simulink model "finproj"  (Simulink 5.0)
settings: Solver=ode45  StartTime=0.0  StopTime=100.0  RelTol=1e-3
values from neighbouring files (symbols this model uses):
  denp = (abs(denp)>1e-8).*denp    [segway.m]
  nump = [nump 0]/numv(2)    [segway.m]

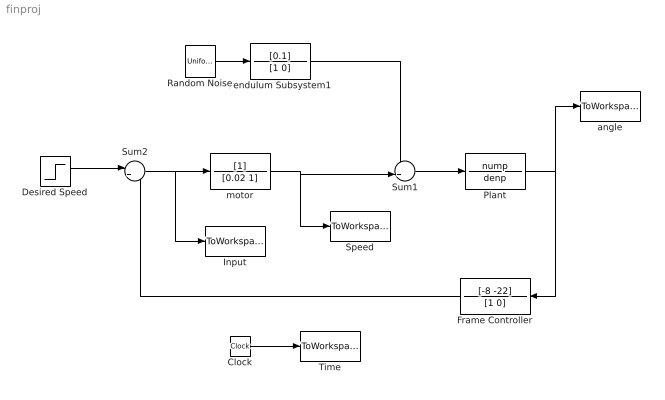
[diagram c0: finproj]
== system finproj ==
  Clock : Clock
  Desired Speed : Step  Time=0  After=0  SampleTime=0
  Frame Controller : TransferFcn  Orientation=left  Numerator=[-8 -22]  Denominator=[1 0]
  Input : ToWorkspace  VariableName=u  SampleTime=-1  SaveFormat=Array
  Pendulum Subsystem1 : TransferFcn  Numerator=[0.1]  Denominator=[1 0]
  Plant : TransferFcn  Numerator=nump  Denominator=denp
  Random Noise : UniformRandomNumber  SampleTime=0
  Speed : ToWorkspace  VariableName=v  SampleTime=-1  SaveFormat=Array
  Sum1 : Sum  Inputs=++|
  Sum2 : Sum  Inputs=|+-
  Time : ToWorkspace  VariableName=t  SampleTime=-1  SaveFormat=Array
  angle : ToWorkspace  VariableName=th  SampleTime=-1  SaveFormat=Array
  motor : TransferFcn  Denominator=[0.02 1]
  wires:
  Plant/1 -> Frame Controller/1, angle/1
  Clock/1 -> Time/1
  Sum2/1 -> motor/1, Input/1
  Desired Speed/1 -> Sum2/1
  Frame Controller/1 -> Sum2/2
  Random Noise/1 -> Pendulum Subsystem1/1
  Pendulum Subsystem1/1 -> Sum1/1
  Sum1/1 -> Plant/1
  motor/1 -> Sum1/2, Speed/1
